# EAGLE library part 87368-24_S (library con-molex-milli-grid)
RECEPTACAL
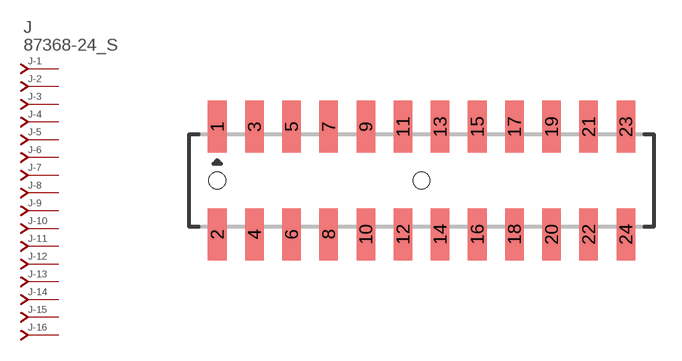
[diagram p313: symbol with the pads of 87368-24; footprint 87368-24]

Designator prefix J; gates -1=J-NV -2=J-N -3=J-N -4=J-N -5=J-N -6=J-N -7=J-N -8=J-N -9=J-N -10=J-N -11=J-N -12=J-N -13=J-N -14=J-N -15=J-N -16=J-N -17=J-N -18=J-N -19=J-N -20=J-N -21=J-N -22=J-N -23=J-N -24=J-N

## 87368-24_S  [87368-24]
1  -1:J  pas
2  -2:J  pas
3  -3:J  pas
4  -4:J  pas
5  -5:J  pas
6  -6:J  pas
7  -7:J  pas
8  -8:J  pas
9  -9:J  pas
10  -10:J  pas
11  -11:J  pas
12  -12:J  pas
13  -13:J  pas
14  -14:J  pas
15  -15:J  pas
16  -16:J  pas
17  -17:J  pas
18  -18:J  pas
19  -19:J  pas
20  -20:J  pas
21  -21:J  pas
22  -22:J  pas
23  -23:J  pas
24  -24:J  pas

## Footprint 87368-24 (pad centres in mm)
RECEPTACAL SMD Dual Row, Side Entry
smd 1 x 2.8: 1 -11,2.9; 2 -11,-2.9; 3 -9,2.9; 4 -9,-2.9; 5 -7,2.9; 6 -7,-2.9; 7 -5,2.9; 8 -5,-2.9; 9 -3,2.9; 10 -3,-2.9; 11 -1,2.9; 12 -1,-2.9; 13 1,2.9; 14 1,-2.9; 15 3,2.9; 16 3,-2.9; 17 5,2.9; 18 5,-2.9; 19 7,2.9; 20 7,-2.9; 21 9,2.9; 22 9,-2.9; 23 11,2.9; 24 11,-2.9
hole 0.914 at -11,0
hole 0.914 at 0,0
